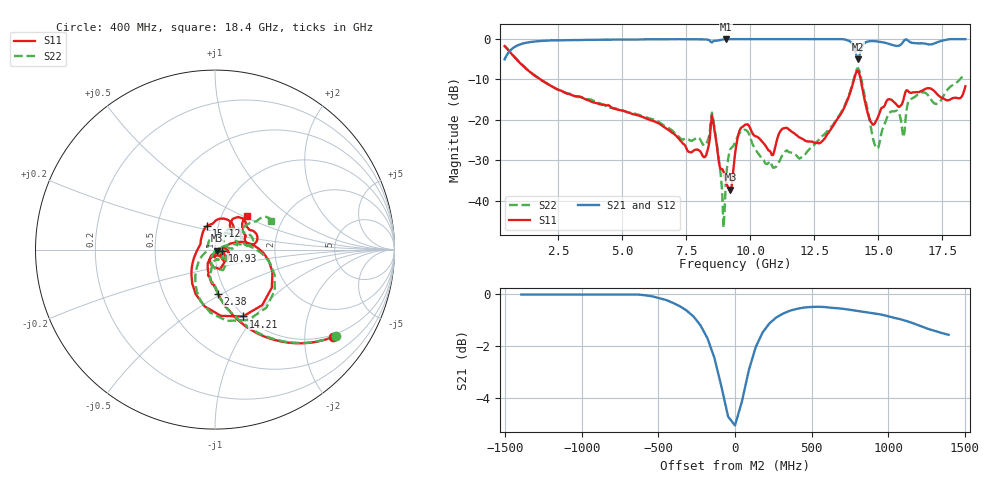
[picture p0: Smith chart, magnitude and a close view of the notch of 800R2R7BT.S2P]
!  American Technical Ceramics  Date:  10/25/10
!  One Norden Lane
!  Huntington Station,  NY.  11746-2102
!  Tel:  (631) 622-4700  Fax:  (631) 622-4748
!  Part Number  800R2R7BT  Mounting Orientation: Vertical
!  Description: Ultra Low ESR Microwave Capacitor
!  Application: Coupling, Bypass, Tuning, DC Block, Filters, Matching
# GHZ S DB R 50
! Freq  |S11|  S11 Ph  |S21|  S21 Ph  |S12|  S12 Ph  |S22|  S22 Ph
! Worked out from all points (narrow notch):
!   401 points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, 400 MHz to 18.4 GHz, reference 50 ohm
!   highest |S21| = 0.00 dB at 9.04 GHz (marker M1); lowest = -5.0 dB at 14.21 GHz (marker M2)
!   notch at M2: 4.9 dB deep, 236 MHz wide at half that depth
!   lowest |S11| = -37.3 dB at 9.22 GHz (marker M3), VSWR 1.03, Z = 51.2 - j0.674 ohm
!   |S11| at or under -10 dB: 1.8 GHz to 14.05 GHz (12.25 GHz wide, 155 % of centre); 14.31 GHz to end of sweep
!   |S22| runs from -46.7 to -1.6 dB; largest |S21 - S12| = 0.0021
!   S11 on the Smith chart (normalised r, x): 400 MHz: 0.93, -2.76; 2.38 GHz: 0.92, -0.48; 10.93 GHz: 1.08, -0.02; 14.21 GHz: 0.98, -0.87; 15.12 GHz: 0.88, +0.24; 18.4 GHz: 1.31, +0.53
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0.4  -1.73 -36.4  -5.03 53.6  -5.03 53.6  -1.63 -35.5
2.38  -12.20 -86.0  -0.31 3.3  -0.31 3.3  -12.21 -86.4
3.415  -14.45 -95.4  -0.20 -4.9  -0.19 -4.9  -14.44 -93.7
6.43  -20.90 -116.9  -0.06 -22.2  -0.06 -22.2  -20.54 -101.1
8.185  -29.25 -78.3  -0.08 -31.9  -0.08 -31.9  -26.33 -65.4
8.545  -20.33 -98.3  -0.55 -30.7  -0.54 -30.8  -19.60 -90.7
8.905  -32.21 -91.4  -0.14 -31.1  -0.13 -31.1  -38.60 -106.6
9.04  -35.15 -79.7  0.00 -31.6  -0.01 -31.6  -35.62 20.2
9.22  -37.31 -28.9  -0.01 -32.7  -0.01 -32.8  -27.20 1.1
9.4  -28.51 14.6  -0.01 -33.2  -0.01 -33.2  -25.60 -3.7
9.805  -21.19 -31.5  -0.01 -37.9  -0.01 -37.9  -22.48 -32.0
10.93  -27.80 -10.6  -0.01 -45.0  -0.01 -45.0  -31.83 -9.6
11.335  -22.04 -20.6  -0.01 -46.6  -0.01 -46.6  -28.08 7.8
12.415  -25.38 -14.7  -0.01 -55.4  -0.01 -55.5  -26.54 19.9
13.81  -14.86 12.3  -0.33 -71.1  -0.32 -71.1  -14.56 6.3
14.215  -7.88 -67.3  -5.05 -60.4  -5.05 -60.4  -7.26 -64.7
14.71  -20.54 175.7  -0.49 -59.8  -0.49 -59.8  -21.93 -154.2
15.115  -17.10 109.5  -0.73 -65.3  -0.72 -65.3  -23.39 111.0
15.43  -14.87 67.9  -1.23 -67.2  -1.22 -67.3  -18.32 45.6
15.97  -15.22 60.7  -0.67 -59.1  -0.68 -59.1  -24.28 21.5
16.285  -13.30 37.0  -0.87 -68.7  -0.85 -68.7  -14.80 34.5
18.4  -11.68 46.6  -0.01 -78.1  -0.01 -78.2  -9.04 27.0
